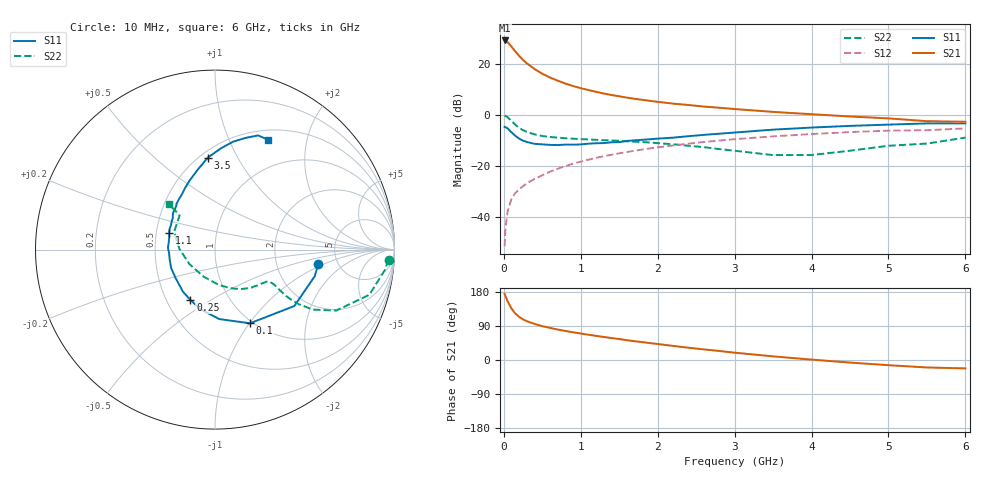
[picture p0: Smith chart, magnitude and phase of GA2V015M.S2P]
! Infineon Technologies  Discrete & RF Semiconductors
! BF775
! Si NPN RF Bipolar Junction Transistor in SOT23
! VCE = 2 V  IC = 15 mA
! Common Emitter S-Parameters:  May  1996
# GHz  S  MA  R  50
!  f  S11  S21  S12  S22
! GHz  MAG  ANG  MAG  ANG  MAG  ANG  MAG  ANG
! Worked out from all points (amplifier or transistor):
!   36 points, 10 MHz to 6 GHz, reference 50 ohm
!   highest |S21| = 29.1 dB at 10 MHz (marker M1)
!   |S21| within 3 dB of that: start of sweep to 115.1 MHz
!   unconditionally stable (mu >= 1): 417.4 MHz to 3.643 GHz
!   at 250 MHz: K = 0.83, MSG = 24.7 dB, |S12| = -27.9 dB
!   at 1.4 GHz: K = 1.13, MAG = 9.5 dB, |S12| = -15.6 dB
!   at 6 GHz: K = 0.98, MSG = 1.3 dB, |S12| = -5.3 dB
!   S11 on the Smith chart (normalised r, x): 10 MHz: 3.56, -0.84; 100 MHz: 0.97, -1.01; 250 MHz: 0.66, -0.41; 1.1 GHz: 0.58, +0.12; 3.5 GHz: 0.55, +0.76; 6 GHz: 0.62, +1.41
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0.01  0.5811 -7.7  28.54 174.5  0.0027 87.9  0.9685 -3.3
0.02  0.5753 -14.9  28.2 169.0  0.0059 85.2  0.9528 -6.9
0.05  0.5424 -35.4  26.44 154.6  0.0132 76.8  0.8963 -16.3
0.1  0.4546 -64.6  21.59 135.7  0.0228 67.3  0.7561 -26.7
0.15  0.3877 -86.5  17.33 122.3  0.0297 63.3  0.64 -31.5
0.2  0.342 -103.8  14.19 113.6  0.035 63.6  0.5575 -33.1
0.25  0.3123 -116.0  11.86 107.2  0.0403 63.2  0.5009 -33.3
0.3  0.2949 -127.2  10.16 102.3  0.0459 64.3  0.4636 -33.0
0.4  0.2707 -144.2  7.865 95.2  0.056 65.9  0.4147 -31.7
0.5  0.2651 -157.0  6.364 89.3  0.0658 66.6  0.3859 -30.7
0.6  0.2589 -166.9  5.378 84.7  0.0775 67.1  0.3697 -30.4
0.7  0.2564 -175.0  4.66 80.4  0.0882 67.1  0.3586 -30.5
0.8  0.2623 177.8  4.093 76.6  0.0994 66.8  0.3491 -30.8
0.9  0.2609 171.2  3.664 73.1  0.1109 66.3  0.3417 -31.4
1.1  0.2732 159.7  3.056 66.7  0.133 65.3  0.3302 -33.9
1.3  0.2805 150.9  2.613 60.8  0.1552 63.4  0.3195 -36.6
1.6  0.3092 139.4  2.17 52.3  0.1878 60.2  0.304 -41.9
2.2  0.3583 121.1  1.658 37.2  0.2525 53.4  0.2662 -55.5
3.5  0.5139 94.5  1.143 9.6  0.3796 35.9  0.1632 -112.9
4.5  0.6089 80.6  0.93 -6.8  0.46 22.2  0.1988 178.6
5.5  0.68 69.3  0.753 -19.7  0.5015 7.7  0.2744 135.8
6  0.6795 64.1  0.732 -22.2  0.5424 3.6  0.3589 135.4
